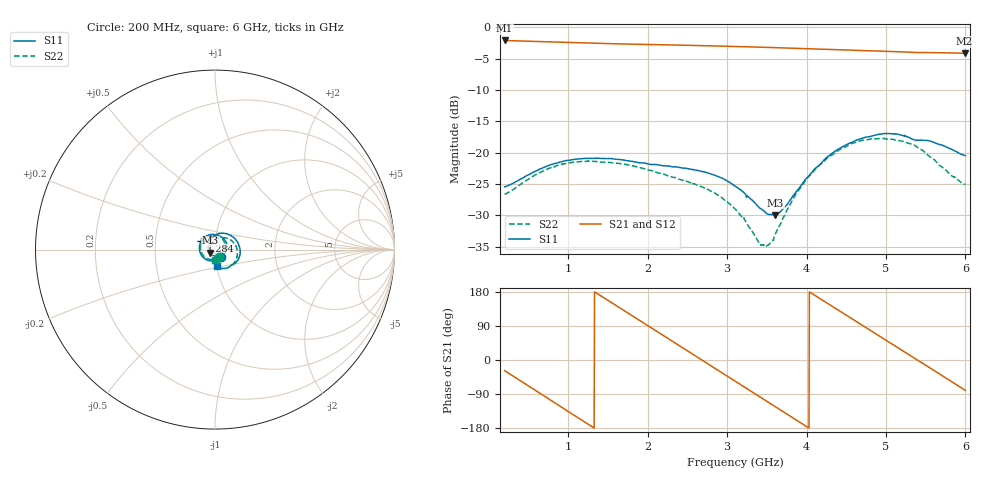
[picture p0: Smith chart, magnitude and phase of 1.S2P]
!Agilent Technologies,E5071C,MY46316741,A.11.02
!Date: Fri Apr 15 16:19:24 2022
!Data & Calibration Information:
!Freq	S11:SOLT2(ON)	S21:SOLT2(ON)	S12:SOLT2(ON)	S22:SOLT2(ON)
!PortZ  Port1:50+j0  Port2:50+j0
!Above PortZ is port z conversion or system Z0 setting when saving the data.
!When reading, reference impedance value at option line is always used.
# Hz S dB R 50
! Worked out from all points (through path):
!   1200 points, 200 MHz to 6 GHz, reference 50 ohm
!   highest |S21| = -2.09 dB at 200 MHz (marker M1); lowest = -4.1 dB at 5.99 GHz (marker M2)
!   group delay of S21, straight-line fit = 370 ps
!   lowest |S11| = -30.0 dB at 3.606 GHz (marker M3), VSWR 1.07, Z = 47.3 - j1.59 ohm
!   |S11| at or under -10 dB: start of sweep to end of sweep
!   |S22| runs from -34.9 to -17.7 dB; largest |S21 - S12| = 0.0024
!   S11 on the Smith chart (normalised r, x): 200 MHz: 1.06, -0.09; 1.284 GHz: 0.86, +0.08; 6 GHz: 1.01, -0.19
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2e8  -25.46 -52.8  -2.09 -28.0  -2.09 -28.0  -26.66 -58.6
4.563803e8  -23.84 -100.6  -2.20 -62.6  -2.20 -62.6  -24.57 -109.6
6.788991e8  -22.44 -135.9  -2.28 -92.6  -2.28 -92.6  -22.97 -146.6
9.062552e8  -21.48 -167.6  -2.36 -123.2  -2.36 -123.1  -21.92 -179.7
1.167473e9  -20.98 160.3  -2.46 -158.2  -2.46 -158.1  -21.42 146.4
1.28357e9  -20.93 147.3  -2.51 -173.7  -2.51 -173.6  -21.41 132.2
1.510926e9  -20.94 123.5  -2.59 156.0  -2.59 156.0  -21.55 107.2
1.757631e9  -21.32 99.7  -2.67 123.3  -2.67 123.3  -21.95 80.9
2.134946e9  -21.96 68.0  -2.77 73.0  -2.77 73.1  -23.23 45.1
2.401001e9  -22.38 44.7  -2.83 37.6  -2.83 37.6  -24.27 22.3
2.628357e9  -22.83 23.3  -2.90 7.3  -2.90 7.3  -25.20 2.4
2.855713e9  -23.67 -1.2  -2.97 -23.1  -2.97 -23.0  -26.51 -20.7
3.102419e9  -25.36 -33.4  -3.05 -56.0  -3.05 -55.9  -29.01 -52.2
3.431359e9  -29.00 -96.9  -3.17 -99.8  -3.17 -99.7  -34.69 -131.1
3.605505e9  -29.95 -148.1  -3.23 -123.0  -3.23 -122.9  -33.08 158.9
3.847373e9  -26.63 144.8  -3.34 -155.2  -3.34 -155.1  -27.06 103.0
4.069892e9  -23.11 102.8  -3.44 175.2  -3.44 175.3  -23.23 70.0
4.577815e9  -18.31 36.0  -3.64 107.9  -3.64 108.0  -18.52 9.2
5.037364e9  -16.96 -13.6  -3.83 47.1  -3.83 47.2  -17.84 -39.7
5.492077e9  -18.03 -50.8  -4.03 -12.7  -4.03 -12.6  -19.98 -80.2
5.990325e9  -20.44 -81.6  -4.15 -78.9  -4.15 -78.9  -25.05 -88.9
6e9  -20.49 -81.8  -4.15 -80.2  -4.16 -80.1  -25.11 -88.5
